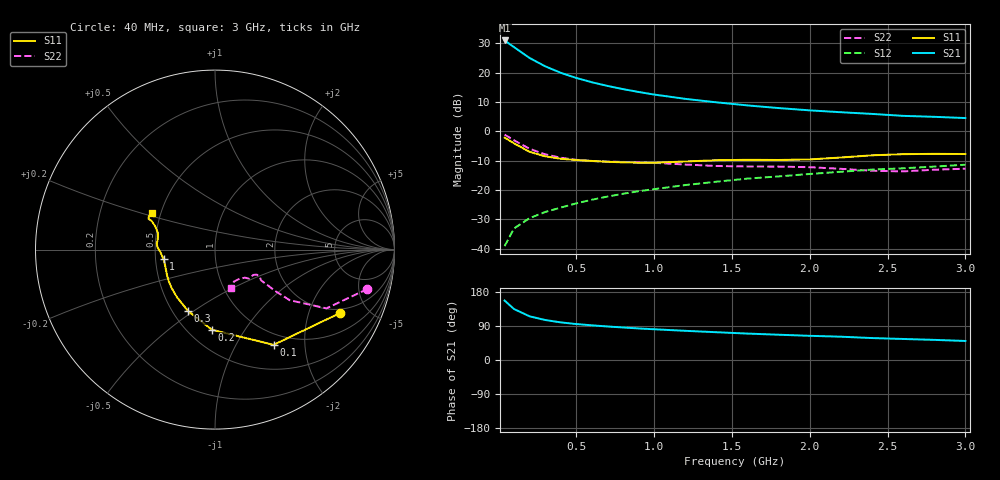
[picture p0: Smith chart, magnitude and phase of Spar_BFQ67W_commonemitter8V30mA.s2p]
! Filename:  BFQ67WL.S2P  Version:  4.0
! NXP part #: BFQ67W  Date: Jun 1994
! Bias condition: Vce=8V, Ic=30mA
#  MHz  S  MA  R  50
! Freq  S11  S21  S12  S22  !GUM [dB]
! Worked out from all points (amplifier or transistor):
!   21 points, 40 MHz to 3 GHz, reference 50 ohm
!   highest |S21| = 31.0 dB at 40 MHz (marker M1)
!   |S21| within 3 dB of that: start of sweep to 120.1 MHz
!   unconditionally stable (mu >= 1): 550.5 MHz to end of sweep
!   at 300 MHz: K = 0.83, MSG = 24.8 dB, |S12| = -27.5 dB
!   at 1 GHz: K = 1.10, MAG = 14.2 dB, |S12| = -19.7 dB
!   at 3 GHz: K = 1.03, MAG = 7.0 dB, |S12| = -11.4 dB
!   lowest NFmin = 2.80 dB at 1 GHz
!   S11 on the Smith chart (normalised r, x): 40 MHz: 1.79, -3.24; 100 MHz: 0.83, -1.44; 200 MHz: 0.65, -0.72; 300 MHz: 0.60, -0.48; 1 GHz: 0.55, -0.07; 3 GHz: 0.44, +0.22
40  0.78 -27.0  35.29 156.9  0.011 76.8  0.877 -14.5
100  0.623 -58.4  27.21 134.6  0.022 65.2  0.702 -27.8
200  0.447 -92.2  17.77 115.3  0.033 61.1  0.503 -34.1
300  0.374 -113.5  12.82 105.6  0.042 62.2  0.405 -34.5
400  0.34 -128.4  9.936 99.3  0.05 64.5  0.354 -34.1
500  0.323 -138.3  8.11 94.9  0.059 66.3  0.326 -33.9
600  0.312 -145.9  6.847 91.5  0.068 67.7  0.311 -33.7
700  0.302 -152.5  5.933 88.5  0.077 69.0  0.304 -33.3
800  0.295 -158.1  5.229 85.8  0.086 70.0  0.3 -32.5
900  0.291 -163.9  4.68 83.3  0.095 70.5  0.295 -31.8
1000  0.291 -169.2  4.226 81.1  0.103 71.0  0.29 -31.1
1200  0.305 -177.5  3.569 77.0  0.121 71.5  0.271 -31.0
1400  0.321 177.7  3.114 73.3  0.138 71.9  0.256 -33.4
1600  0.326 173.9  2.758 69.7  0.156 71.3  0.251 -37.7
1800  0.324 169.7  2.485 66.7  0.17 71.6  0.25 -40.3
2000  0.331 163.8  2.27 63.8  0.187 71.6  0.244 -41.2
2200  0.357 158.8  2.111 61.5  0.204 71.9  0.229 -43.1
2400  0.389 155.5  1.975 57.9  0.222 71.5  0.212 -50.2
2600  0.407 155.3  1.83 55.5  0.234 70.7  0.207 -59.3
2800  0.412 153.8  1.762 53.1  0.25 70.9  0.221 -64.9
3000  0.409 149.8  1.679 50.2  0.269 70.5  0.23 -67.5
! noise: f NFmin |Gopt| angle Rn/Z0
1000  2.8  0.23  97  0.332
